| TEXAS INSTRUMENTS INCORPORATED
| Standard Linear and Logic Group
| IBIS Model of SN74LV373AT
| OCTAL TRANSPARENT D-TYPE LATCH WITH 3-STATE OUTPUT
| This file contains package information for the following:
|  SOIC 20-pin (DW) package as [Component] LV373AT_DW
|  SSOP 20-pin (DB) package as [Component] LV373AT_DB
|  TSSOP 20-pin (PW) package as [Component] LV373AT_PW
|  QFN 20-pin (RGY) package as [Component] LV373AT_RGY
|  SOP 20-pin (NS) package as [Component] LV373AT_NS
| This device can be powered at the following Vccs:
|  5 volt Vcc
| This file provides unique models under the [Model Selector] for each Vcc.
| For operation at a specific Vcc, select the appropriate model after each
| [Model Selector] keyword.
[IBIS Ver]   3.2
[Comment char]  |_char
[File Name]   sn74lv373at.ibs
[File Rev]   1.1 | x_die
[Date]   August 4, 2005
[Source]   Data created from TI-SPICE simulations at TI-SLL.
[Notes]   The following is an IBIS list for the LV373AT.
   Please contact sllibis@ti.com with questions and
   comments concerning SLL IBIS models.
   - FILE REV HISTORY
   - 1.1 Release IBIS file on 08/19/05
   - Non-monotonic data in pullup due to Ioff circuitry at output.
   - Power clamp data deleted as there is no power-clamp diode.
   - C_comp values for the input models have been replaced
   by the data sheet values.
[Disclaimer] Property of Texas Instruments Incorporated.  Unauthorized
   reproduction and/or distribution is strictly prohibited.
   This product is protected under copyright law.
   Created  2005, (C) Copyright  2005, Texas Instruments
   Incorporated, All Rights Reserved
   UNLESS THERE IS A SIGNED, WRITTEN AGREEMENT TO THE
   CONTRARY, TEXAS INSTRUMENTS (TI) IS PROVIDING THE IBIS
   MODELS  AND WITHOUT ANY WARRANTY, EXPRESSED OR
   IMPLIED.  TI assumes no liability for:
   1) the accuracy of the IBIS models provided to your
   company;
   2) the proper functioning of these IBIS Models in your
   design or for any resulting applications; or
   3) infringement of patents, copyrights or intellectual
   property rights resulting from your use of these IBIS
   models.
   TI provides IBIS Models as a service to our customers.
   You and your company shall not distribute, sell or give
   these models to anyone else without prior written
   permission from TI.
   TI reserves the right to make changes to our products or
   to discontinue any semiconductor product or service
   without notice, and advises our customers to obtain the
   latest version of relevant information to verify, before
   placing orders, that the information being relied on is
   current.
   Please be aware that your receipt and use of the IBIS
   information provided shall serve as acceptance of these
   terms and conditions.  If you do not accept these terms,
   you should return or destroy the IBIS models and any
   other accompanying information immediately.
| Component LV373AT_DW 20-pin SOIC
[Component]   LV373AT_DW
[Manufacturer]   Texas Instruments, Inc.
[Package]
|   typ   min   max
R_pkg   3.800e-02   3.300e-02   4.500e-02
L_pkg   5.012e-09   4.110e-09   6.349e-09
C_pkg   7.170e-13   5.300e-13   8.680e-13
[Pin]   signal_name   model_name   R_pin   L_pin   C_pin
1   NOE   LV373AT_IN   4.200e-02   6.336e-09   8.650e-13
2   1Q   LV373AT_OUT   4.300e-02   5.542e-09   8.670e-13
3   1D   LV373AT_IN   3.400e-02   4.714e-09   7.320e-13
4   2D   LV373AT_IN   3.400e-02   4.377e-09   5.910e-13
5   2Q   LV373AT_OUT   3.600e-02   4.130e-09   5.330e-13
6   3Q   LV373AT_OUT   3.500e-02   4.111e-09   5.300e-13
7   3D   LV373AT_IN   3.400e-02   4.284e-09   5.830e-13
8   4D   LV373AT_IN   3.400e-02   4.634e-09   7.260e-13
9   4Q   LV373AT_OUT   4.000e-02   5.518e-09   8.650e-13
10   GND   GND   4.300e-02   6.349e-09   8.660e-13
11   LE   LV373AT_IN   4.100e-02   6.281e-09   8.610e-13
12   5Q   LV373AT_OUT   4.500e-02   5.561e-09   8.680e-13
13   5D   LV373AT_IN   3.300e-02   4.778e-09   7.420e-13
14   6D   LV373AT_IN   3.500e-02   4.414e-09   5.960e-13
15   6Q   LV373AT_OUT   3.500e-02   4.110e-09   5.330e-13
16   7Q   LV373AT_OUT   3.600e-02   4.130e-09   5.330e-13
17   7D   LV373AT_IN   3.400e-02   4.377e-09   5.910e-13
18   8D   LV373AT_IN   3.400e-02   4.714e-09   7.310e-13
19   8Q   LV373AT_OUT   4.300e-02   5.569e-09   8.680e-13
20   VCC   POWER   4.200e-02   6.308e-09   8.640e-13
| Component LV373AT_DB 20-pin SSOP
[Component]   LV373AT_DB
[Manufacturer]   Texas Instruments, Inc.
[Package]
|   typ   min   max
R_pkg   4.000e-02   3.500e-02   5.100e-02
L_pkg   3.495e-09   3.035e-09   4.314e-09
C_pkg   4.200e-13   3.460e-13   5.020e-13
[Pin]   signal_name   model_name   R_pin   L_pin   C_pin
1   NOE   LV373AT_IN   4.900e-02   4.310e-09   5.020e-13
2   1Q   LV373AT_OUT   4.800e-02   3.903e-09   4.870e-13
3   1D   LV373AT_IN   3.500e-02   3.189e-09   3.960e-13
4   2D   LV373AT_IN   3.500e-02   3.036e-09   3.470e-13
5   2Q   LV373AT_OUT   3.500e-02   3.035e-09   3.670e-13
6   3Q   LV373AT_OUT   3.500e-02   3.035e-09   3.670e-13
7   3D   LV373AT_IN   3.500e-02   3.036e-09   3.470e-13
8   4D   LV373AT_IN   3.500e-02   3.189e-09   3.970e-13
9   4Q   LV373AT_OUT   4.700e-02   3.899e-09   4.880e-13
10   GND   GND   5.100e-02   4.314e-09   5.000e-13
11   LE   LV373AT_IN   5.100e-02   4.314e-09   5.000e-13
12   5Q   LV373AT_OUT   4.700e-02   3.899e-09   4.880e-13
13   5D   LV373AT_IN   3.500e-02   3.189e-09   3.970e-13
14   6D   LV373AT_IN   3.500e-02   3.036e-09   3.460e-13
15   6Q   LV373AT_OUT   3.500e-02   3.035e-09   3.670e-13
16   7Q   LV373AT_OUT   3.500e-02   3.035e-09   3.670e-13
17   7D   LV373AT_IN   3.500e-02   3.036e-09   3.460e-13
18   8D   LV373AT_IN   3.500e-02   3.189e-09   3.970e-13
19   8Q   LV373AT_OUT   4.700e-02   3.899e-09   4.880e-13
20   VCC   POWER   5.100e-02   4.314e-09   5.020e-13
| Component LV373AT_PW 20-pin TSSOP
[Component]   LV373AT_PW
[Manufacturer]   Texas Instruments, Inc.
[Package]
|   typ   min   max
R_pkg   4.500e-02   3.600e-02   5.700e-02
L_pkg   2.694e-09   2.290e-09   3.177e-09
C_pkg   1.560e-13   7.600e-14   2.590e-13
[Pin]   signal_name   model_name   R_pin   L_pin   C_pin
1   NOE   LV373AT_IN   3.600e-02   3.045e-09   2.590e-13
2   1Q   LV373AT_OUT   5.100e-02   3.013e-09   1.890e-13
3   1D   LV373AT_IN   4.400e-02   2.695e-09   1.640e-13
4   2D   LV373AT_IN   4.700e-02   2.362e-09   7.900e-14
5   2Q   LV373AT_OUT   4.700e-02   2.333e-09   8.600e-14
6   3Q   LV373AT_OUT   4.700e-02   2.298e-09   8.500e-14
7   3D   LV373AT_IN   4.700e-02   2.351e-09   7.900e-14
8   4D   LV373AT_IN   4.400e-02   2.706e-09   1.650e-13
9   4Q   LV373AT_OUT   4.900e-02   2.999e-09   1.880e-13
10   GND   GND   3.900e-02   3.039e-09   2.570e-13
11   LE   LV373AT_IN   3.800e-02   3.044e-09   2.580e-13
12   5Q   LV373AT_OUT   5.700e-02   3.177e-09   1.990e-13
13   5D   LV373AT_IN   4.400e-02   2.825e-09   1.730e-13
14   6D   LV373AT_IN   4.700e-02   2.429e-09   8.300e-14
15   6Q   LV373AT_OUT   4.900e-02   2.383e-09   9.000e-14
16   7Q   LV373AT_OUT   4.900e-02   2.347e-09   8.900e-14
17   7D   LV373AT_IN   4.700e-02   2.290e-09   7.600e-14
18   8D   LV373AT_IN   4.500e-02   2.613e-09   1.580e-13
19   8Q   LV373AT_OUT   4.400e-02   2.883e-09   1.810e-13
20   VCC   POWER   3.900e-02   3.044e-09   2.560e-13
| Component LV373AT_NS 20-pin SOP
[Component]   LV373AT_NS
[Manufacturer]   Texas Instruments, Inc.
[Package]
|   typ   min   max
R_pkg   4.400e-02   2.900e-02   5.800e-02
L_pkg   3.666e-09   2.317e-09   5.115e-09
C_pkg   5.480e-13   3.160e-13   7.250e-13
[Pin]   signal_name   model_name   R_pin   L_pin   C_pin
1   NOE   LV373AT_IN   5.800e-02   5.115e-09   7.250e-13
2   1Q   LV373AT_OUT   5.300e-02   4.591e-09   7.240e-13
3   1D   LV373AT_IN   4.900e-02   3.754e-09   5.720e-13
4   2D   LV373AT_IN   2.900e-02   2.549e-09   3.880e-13
5   2Q   LV373AT_OUT   3.100e-02   2.317e-09   3.160e-13
6   3Q   LV373AT_OUT   3.100e-02   2.317e-09   3.160e-13
7   3D   LV373AT_IN   2.900e-02   2.556e-09   3.990e-13
8   4D   LV373AT_IN   4.900e-02   3.754e-09   5.790e-13
9   8Q   LV373AT_OUT   5.300e-02   4.591e-09   7.240e-13
10   GND   GND   5.800e-02   5.115e-09   7.250e-13
11   LE   LV373AT_IN   5.800e-02   5.115e-09   7.250e-13
12   5Q   LV373AT_OUT   5.300e-02   4.591e-09   7.240e-13
13   5D   LV373AT_IN   4.900e-02   3.754e-09   5.790e-13
14   6D   LV373AT_IN   2.900e-02   2.557e-09   3.990e-13
15   6Q   LV373AT_OUT   3.100e-02   2.317e-09   3.160e-13
16   7Q   LV373AT_OUT   3.100e-02   2.317e-09   3.160e-13
17   7D   LV373AT_IN   2.900e-02   2.557e-09   3.990e-13
18   8D   LV373AT_IN   4.900e-02   3.754e-09   5.790e-13
19   8Q   LV373AT_OUT   5.300e-02   4.591e-09   7.240e-13
20   VCC   POWER   5.800e-02   5.115e-09   7.250e-13
| Component LV373AT_RGY 20-pin QFN
[Component]   LV373AT_RGY
[Manufacturer]   Texas Instruments, Inc.
[Package]
|   typ   min   max
R_pkg   0.046   0.035   0.058
L_pkg   1.131nH   0.880nH   1.396nH
C_pkg   0.165pF   0.142pF   0.175pF
[Pin]   signal_name   model_name   R_pin   L_pin   C_pin
1   NOE   LV373AT_IN   0.053   1.289nH   0.142pF
2   1Q   LV373AT_OUT   0.058   1.386nH   0.172pF
3   1D   LV373AT_IN   0.046   1.111nH   0.173pF
4   2D   LV373AT_IN   0.039   0.965nH   0.161pF
5   2Q   LV373AT_OUT   0.035   0.881nH   0.165pF
6   3Q   LV373AT_OUT   0.035   0.880nH   0.165pF
7   3D   LV373AT_IN   0.039   0.961nH   0.161pF
8   4D   LV373AT_IN   0.045   1.105nH   0.172pF
9   4Q   LV373AT_OUT   0.058   1.386nH   0.172pF
10   GND   GND   0.056   1.352nH   0.159pF
11   LE   LV373AT_IN   0.053   1.287nH   0.155pF
12   5Q   LV373AT_OUT   0.058   1.396nH   0.172pF
13   5D   LV373AT_IN   0.047   1.129nH   0.175pF
14   6D   LV373AT_IN   0.040   0.976nH   0.164pF
15   6Q   LV373AT_OUT   0.035   0.884nH   0.169pF
16   7Q   LV373AT_OUT   0.035   0.881nH   0.168pF
17   7D   LV373AT_IN   0.039   0.967nH   0.162pF
18   8D   LV373AT_IN   0.046   1.118nH   0.174pF
19   8Q   LV373AT_OUT   0.058   1.396nH   0.175pF
20   VCC   POWER   0.052   1.276nH   0.144pF
| Model LV373AT_IN
[Model Selector]   LV373AT_IN
LV373AT_IN_50_85C   5 volt Vcc
LV373AT_IN_50_125C   5 volt Vcc
| Model LV373AT_OUT
[Model Selector]   LV373AT_OUT
LV373AT_OUT_50_85C   5 volt Vcc
LV373AT_OUT_50_125C   5 volt Vcc
| Models and submodels in the file (4): LV373AT_IN_50_85C (Input), LV373AT_OUT_50_85C (3-state), LV373AT_IN_50_125C (Input), LV373AT_OUT_50_125C (3-state)
